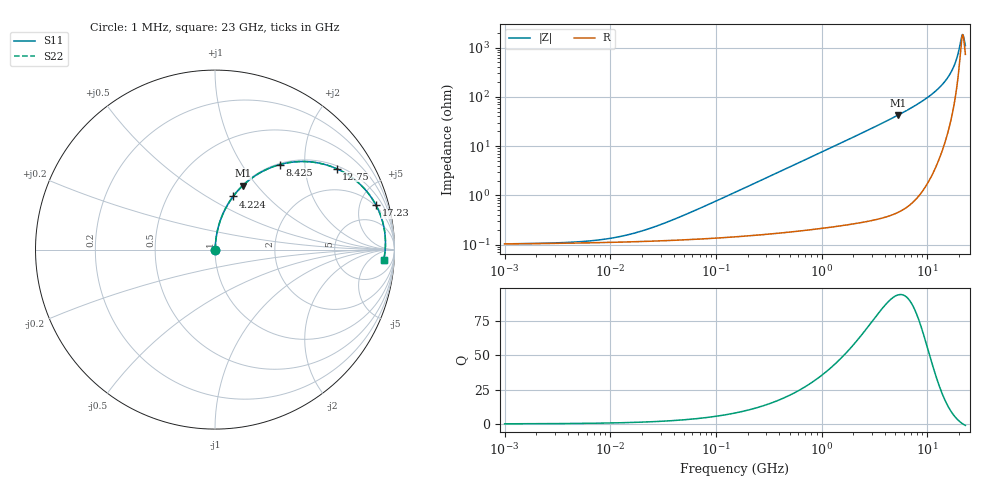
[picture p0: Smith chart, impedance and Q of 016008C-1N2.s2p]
# MHz S MA R 50
!Freq  MagS11  AngS11  MagS21  AngS21  MagS12  AngS12  MagS22  AngS22
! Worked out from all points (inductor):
!   801 points, 1 MHz to 23 GHz, reference 50 ohm
!   read as one part in series: L = 1.2 nH near 50.24 MHz
!   highest Q = 94.1 at 5.295 GHz (marker M1), where L = 1.28 nH
!   self-resonance near 21.74 GHz
!   S11 on the Smith chart (normalised r, x): 1 MHz: 1.00, +0.00; 4.224 GHz: 1.01, +0.66; 8.425 GHz: 1.02, +1.50; 12.75 GHz: 1.10, +2.93; 17.23 GHz: 1.87, +6.91; 23 GHz: 16, -16
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1  0.001037 4.2  0.999 -0.0  0.999 -0.0  0.001037 4.2
5.377611  0.001155 20.5  0.9989 -0.0  0.9989 -0.0  0.001155 20.5
12.78758  0.001482 40.5  0.9989 -0.1  0.9989 -0.1  0.001482 40.5
18.87146  0.001831 50.8  0.9988 -0.1  0.9988 -0.1  0.001831 50.8
28.55793  0.002458 60.9  0.9988 -0.1  0.9988 -0.1  0.002458 60.9
55.5509  0.00437 72.9  0.9987 -0.2  0.9987 -0.2  0.00437 72.9
151.6575  0.01151 82.2  0.9985 -0.7  0.9985 -0.7  0.01151 82.2
815.5551  0.06137 84.6  0.9961 -3.5  0.9961 -3.5  0.06137 84.6
1988.642  0.1492 80.4  0.9862 -8.6  0.9862 -8.6  0.1492 80.4
4223.634  0.3132 71.1  0.9462 -18.3  0.9462 -18.3  0.3132 71.1
4331.024  0.321 70.6  0.9435 -18.7  0.9435 -18.7  0.321 70.6
5294.502  0.3893 66.5  0.917 -22.9  0.917 -22.9  0.3893 66.5
6720.726  0.4868 60.2  0.8682 -29.1  0.8682 -29.1  0.4868 60.2
8424.712  0.5953 52.7  0.7956 -36.5  0.7956 -36.5  0.5953 52.7
10560.73  0.715 43.2  0.6849 -45.6  0.6849 -45.6  0.715 43.2
12749.01  0.8138 33.6  0.5543 -54.4  0.5543 -54.4  0.8138 33.6
15198.7  0.8919 23.4  0.3972 -62.9  0.3972 -62.9  0.8919 23.4
17231.7  0.9308 15.4  0.2671 -67.4  0.2671 -67.4  0.9308 15.4
18814.53  0.9464 9.6  0.1711 -67.0  0.1711 -67.0  0.9464 9.6
21065.06  0.9505 2.1  0.06081 -34.5  0.06081 -34.5  0.9505 2.1
21873.55  0.9478 -0.4  0.0527 7.4  0.0527 7.4  0.9478 -0.4
23000  0.941 -3.7  0.08588 44.8  0.08588 44.8  0.941 -3.7
